| IBIS file stm32g030_031_041_lqfp48.ibs
[IBIS ver] 4.2
[File name] stm32g030_031_041_lqfp48.ibs
[File Rev] rev1.1
[Date]  12-05-2022
[Source] Data Created at STMicroelectronics
[Notes]  File originated from ELDO simulations.
[Disclaimer]  This information is for modeling purpose only and is
   not guaranted. The information is subject to change without
   notice.
[Copyright] Copyright 2022 STMicroelectronics Inc.
|   Component stm32g030_031_041_lqfp48
[Component] stm32g030_031_041_lqfp48
[Manufacturer] STMicroelectronics
[Package]
| variable   typ   min   max
R_pkg   0.0   0.0   0.0
L_pkg   0.0H   0.0H   0.0H
C_pkg   0.0F   0.0F   0.0F
[Pin]   signal_name   model_name  R_pin L_pin C_pin
1 PC13 io8prog2m25m50m120m_sudq_ft 0.053 3.42534E-09 9.041E-14
2 PC14-OSC32_IN io8prog2m25m50m120m_sudq_ft 0.048377332 2.91404E-09 6.443E-14
3 PC15-OSC32_OUT io8prog2m25m50m120m_sudq_ft 0.044678997 2.50442E-09 4.365E-14
4 VBAT POWER 0.041905328 2.19704E-09 2.807E-14
5 VREF+ POWER 0.040056325 1.9919E-09 1.769E-14
6 VDDA POWER 0.03913 1.89021E-09 1.24625E-14
7 VSS GND 0.03913 1.89021E-09 1.24625E-14
8 PF0-OSC_IN io6_ft 0.040057312 1.98992E-09 1.775E-14
9 PF1-OSC_OUT io6_ft 0.041906973 2.19374E-09 2.817E-14
10 PF2-NRST io6reset 0.0446813 2.4998E-09 4.379E-14
11 PA0 io6_ft 0.048380293 2.9081E-09 6.461E-14
12 PA1 io6_ft 0.053 3.42534E-09 9.041E-14
13 PA2 io6_ft 0.053 3.42534E-09 9.041E-14
14 PA3 io6_ft 0.048377332 2.91404E-09 6.443E-14
15 PA4 io6_ft 0.044678997 2.50442E-09 4.365E-14
16 PA5 io6_ft 0.041905328 2.19704E-09 2.807E-14
17 PA6 io6_ft 0.040056325 1.9919E-09 1.769E-14
18 PA7 io6_ft 0.03913 1.89021E-09 1.24625E-14
19 PB0 io6_ft 0.03913 1.89021E-09 1.24625E-14
20 PB1 io6_ft 0.040057312 1.98992E-09 1.775E-14
21 PB2 io6_ft 0.041906973 2.19374E-09 2.817E-14
22 PB10 io6_i2c_ft 0.0446813 2.4998E-09 4.379E-14
23 PB11 io6_i2c_ft 0.048380293 2.9081E-09 6.461E-14
24 PB12 io6_ft 0.053 3.42534E-09 9.041E-14
25 PB13 io6_i2c_ft 0.053 3.42534E-09 9.041E-14
26 PB14 io6_i2c_ft 0.048377332 2.91404E-09 6.443E-14
27 PB15 io6_ft 0.044678997 2.50442E-09 4.365E-14
28 PA8 io6_ft 0.041905328 2.19704E-09 2.807E-14
29 PA9 io6_i2c_ft 0.040056325 1.9919E-09 1.769E-14
30 PC6 io6_ft 0.03913 1.89021E-09 1.24625E-14
31 PC7 io6_ft 0.03913 1.89021E-09 1.24625E-14
32 PA10 io6_i2c_ft 0.040057312 1.98992E-09 1.775E-14
33 PA11 io6_i2c_ft 0.041906973 2.19374E-09 2.817E-14
34 PA12 io6_i2c_ft 0.0446813 2.4998E-09 4.379E-14
35 PA13 io6_ft 0.048380293 2.9081E-09 6.461E-14
36 PA14-BOOT0 io6_ft 0.053 3.42534E-09 9.041E-14
37 PA15 io6_ft 0.053 3.42534E-09 9.041E-14
38 PD0 io6_ft 0.048377332 2.91404E-09 6.443E-14
39 PD1 io6_ft 0.044678997 2.50442E-09 4.365E-14
40 PD2 io6_ft 0.041905328 2.19704E-09 2.807E-14
41 PD3 io6_ft 0.040056325 1.9919E-09 1.769E-14
42 PB3 io6_ft 0.03913 1.89021E-09 1.24625E-14
43 PB4 io6_ft 0.03913 1.89021E-09 1.24625E-14
44 PB5 io6_ft 0.040057312 1.98992E-09 1.775E-14
45 PB6 io6_i2c_ft 0.041906973 2.19374E-09 2.817E-14
46 PB7 io6_i2c_ft 0.0446813 2.4998E-09 4.379E-14
47 PB8 io6_i2c_ft 0.048380293 2.9081E-09 6.461E-14
48 PB9 io6_i2c_ft 0.053 3.42534E-09 9.041E-14
[Model Selector] io8prog2m25m50m120m_sudq_ft
iols8p_sudq_ft_pd_lv  "IO low speed, PD=40kOhm - 1P8V"
iols8p_sudq_ft_pu_lv  "IO low speed, PU=40kOhm - 1P8V"
iols8p_sudq_ft_lv  "IO low speed - 1P8V"
iols8p_sudq_ft_pd  "IO low speed, PD=40kOhm - 3P3V"
iols8p_sudq_ft_pu  "IO low speed, PU=40kOhm - 3P3V"
iols8p_sudq_ft  "IO low speed - 3P3V"
iofs8p_sudq_ft_pd_lv  "IO full speed, PD=40kOhm - 1P8V"
iofs8p_sudq_ft_pu_lv  "IO full speed, PU=40kOhm - 1P8V"
iofs8p_sudq_ft_lv  "IO full speed - 1P8V"
iofs8p_sudq_ft_pd  "IO full speed, PD=40kOhm - 3P3V"
iofs8p_sudq_ft_pu  "IO full speed, PU=40kOhm - 3P3V"
iofs8p_sudq_ft  "IO full speed - 3P3V"
ioms8p_sudq_ft_pd_lv  "IO medium speed, PD=40kOhm - 1P8V"
ioms8p_sudq_ft_pu_lv  "IO medium speed, PU=40kOhm - 1P8V"
ioms8p_sudq_ft_lv  "IO medium speed - 1P8V"
ioms8p_sudq_ft_pd  "IO medium speed, PD=40kOhm - 3P3V"
ioms8p_sudq_ft_pu  "IO medium speed, PU=40kOhm - 3P3V"
ioms8p_sudq_ft  "IO medium speed - 3P3V"
iohs8p_sudq_ft_pd_lv  "IO high speed, PD=40kOhm - 1P8V"
iohs8p_sudq_ft_pu_lv  "IO high speed, PU=40kOhm - 1P8V"
iohs8p_sudq_ft_lv  "IO high speed - 1P8V"
iohs8p_sudq_ft_pd  "IO high speed, PD=40kOhm - 3P3V"
iohs8p_sudq_ft_pu  "IO high speed, PU=40kOhm - 3P3V"
iohs8p_sudq_ft  "IO high speed - 3P3V"
[Model Selector] io6_ft
io6_ft_1v8_highspeed_pd  "GPIO-1.8V range - high speed - pull down"
io6_ft_1v8_fastspeed_pd  "GPIO-1.8V range - fast speed - pull down"
io6_ft_1v8_mediumspeed_pd  "GPIO-1.8V range - medium speed - pull down"
io6_ft_1v8_lowspeed_pd  "GPIO-1.8V range - low speed - pull down"
io6_ft_1v8_highspeed_pu  "GPIO-1.8V range - high speed - pull up"
io6_ft_1v8_fastspeed_pu  "GPIO-1.8V range - fast speed - pull up"
io6_ft_1v8_mediumspeed_pu  "GPIO-1.8V range - medium speed - pull up"
io6_ft_1v8_lowspeed_pu  "GPIO-1.8V range - low speed - pull up"
io6_ft_1v8_highspeed  "GPIO-1.8V range - high speed"
io6_ft_1v8_fastspeed  "GPIO-1.8V range - fast speed"
io6_ft_1v8_mediumspeed  "GPIO-1.8V range - medium speed"
io6_ft_1v8_lowspeed  "GPIO-1.8V range - low speed"
io6_ft_3v3_highspeed_pd  "GPIO-3.3V range - high speed - pull down"
io6_ft_3v3_fastspeed_pd  "GPIO-3.3V range - fast speed - pull down"
io6_ft_3v3_mediumspeed_pd  "GPIO-3.3V range - medium speed - pull down"
io6_ft_3v3_lowspeed_pd  "GPIO-3.3V range - low speed - pull down"
io6_ft_3v3_highspeed_pu  "GPIO-3.3V range - high speed - pull up"
io6_ft_3v3_fastspeed_pu  "GPIO-3.3V range - fast speed - pull up"
io6_ft_3v3_mediumspeed_pu  "GPIO-3.3V range - medium speed - pull up"
io6_ft_3v3_lowspeed_pu  "GPIO-3.3V range - low speed - pull up"
io6_ft_3v3_highspeed  "GPIO-3.3V range - high speed"
io6_ft_3v3_fastspeed  "GPIO-3.3V range - fast speed"
io6_ft_3v3_mediumspeed  "GPIO-3.3V range - medium speed"
io6_ft_3v3_lowspeed  "GPIO-3.3V range - low speed"
[Model Selector] io6_i2c_ft
io6_ft_1v8_highspeed_pd  "GPIO-1.8V range - high speed - pull down"
io6_ft_1v8_fastspeed_pd  "GPIO-1.8V range - fast speed - pull down"
io6_ft_1v8_mediumspeed_pd  "GPIO-1.8V range - medium speed - pull down"
io6_ft_1v8_lowspeed_pd  "GPIO-1.8V range - low speed - pull down"
io6_ft_1v8_highspeed_pu  "GPIO-1.8V range - high speed - pull up"
io6_ft_1v8_fastspeed_pu  "GPIO-1.8V range - fast speed - pull up"
io6_ft_1v8_mediumspeed_pu  "GPIO-1.8V range - medium speed - pull up"
io6_ft_1v8_lowspeed_pu  "GPIO-1.8V range - low speed - pull up"
io6_ft_1v8_highspeed  "GPIO-1.8V range - high speed"
io6_ft_1v8_fastspeed  "GPIO-1.8V range - fast speed"
io6_ft_1v8_mediumspeed  "GPIO-1.8V range - medium speed"
io6_ft_1v8_lowspeed  "GPIO-1.8V range - low speed"
io6_ft_3v3_highspeed_pd  "GPIO-3.3V range - high speed - pull down"
io6_ft_3v3_fastspeed_pd  "GPIO-3.3V range - fast speed - pull down"
io6_ft_3v3_mediumspeed_pd  "GPIO-3.3V range - medium speed - pull down"
io6_ft_3v3_lowspeed_pd  "GPIO-3.3V range - low speed - pull down"
io6_ft_3v3_highspeed_pu  "GPIO-3.3V range - high speed - pull up"
io6_ft_3v3_fastspeed_pu  "GPIO-3.3V range - fast speed - pull up"
io6_ft_3v3_mediumspeed_pu  "GPIO-3.3V range - medium speed - pull up"
io6_ft_3v3_lowspeed_pu  "GPIO-3.3V range - low speed - pull up"
io6_ft_3v3_highspeed  "GPIO-3.3V range - high speed"
io6_ft_3v3_fastspeed  "GPIO-3.3V range - fast speed"
io6_ft_3v3_mediumspeed  "GPIO-3.3V range - medium speed"
io6_ft_3v3_lowspeed  "GPIO-3.3V range - low speed"
io6_ft_1v8_highi2c_pd   "GPIO-1.8V range - high   speed i2c mode - pd"
io6_ft_1v8_fasti2c_pd   "GPIO-1.8V range - fast   speed i2c mode - pd"
io6_ft_1v8_mediumi2c_pd  "GPIO-1.8V range - medium speed i2c mode - pd"
io6_ft_1v8_lowi2c_pd   "GPIO-1.8V range - low   speed i2c mode - pd"
io6_ft_1v8_highi2c_pu   "GPIO-1.8V range - high   speed i2c mode - pu"
io6_ft_1v8_fasti2c_pu   "GPIO-1.8V range - fast   speed i2c mode - pu"
io6_ft_1v8_mediumi2c_pu  "GPIO-1.8V range - medium speed i2c mode - pu"
io6_ft_1v8_lowi2c_pu   "GPIO-1.8V range - low   speed i2c mode - pu"
io6_ft_1v8_highi2c   "GPIO-1.8V range - high   speed i2c mode"
io6_ft_1v8_fasti2c   "GPIO-1.8V range - fast   speed i2c mode"
io6_ft_1v8_mediumi2c   "GPIO-1.8V range - medium speed i2c mode"
io6_ft_1v8_lowi2c   "GPIO-1.8V range - low   speed i2c mode"
io6_ft_3v3_highi2c_pd   "GPIO-3.3V range - high   speed i2c mode - pd"
io6_ft_3v3_fasti2c_pd   "GPIO-3.3V range - fast   speed i2c mode - pd"
io6_ft_3v3_mediumi2c_pd  "GPIO-3.3V range - medium speed i2c mode - pd"
io6_ft_3v3_lowi2c_pd   "GPIO-3.3V range - low   speed i2c mode - pd"
io6_ft_3v3_highi2c_pu   "GPIO-3.3V range - high   speed i2c mode - pu"
io6_ft_3v3_fasti2c_pu   "GPIO-3.3V range - fast   speed i2c mode - pu"
io6_ft_3v3_mediumi2c_pu  "GPIO-3.3V range - medium speed i2c mode - pu"
io6_ft_3v3_lowi2c_pu   "GPIO-3.3V range - low   speed i2c mode - pu"
io6_ft_3v3_highi2c   "GPIO-3.3V range - high   speed i2c mode"
io6_ft_3v3_fasti2c   "GPIO-3.3V range - fast   speed i2c mode"
io6_ft_3v3_mediumi2c   "GPIO-3.3V range - medium speed i2c mode"
io6_ft_3v3_lowi2c   "GPIO-3.3V range - low   speed i2c mode"
io6_i2c_ft_1v8_pd  "GPIO-1.8V I2C fm+ - pd"
io6_i2c_ft_3v3_pd  "GPIO-3.3V I2C fm+ - pd"
io6_i2c_ft_1v8_pu  "GPIO-1.8V I2C fm+ - pu"
io6_i2c_ft_3v3_pu  "GPIO-3.3V I2C fm+ - pu"
io6_i2c_ft_1v8   "GPIO-1.8V I2C fm+"
io6_i2c_ft_3v3   "GPIO-3.3V I2C fm+"
[Model Selector] io6reset
io6_ft_1v8_highspeed_pd  "GPIO-1.8V range - high speed - pull down"
io6_ft_1v8_fastspeed_pd  "GPIO-1.8V range - fast speed - pull down"
io6_ft_1v8_mediumspeed_pd  "GPIO-1.8V range - medium speed - pull down"
io6_ft_1v8_lowspeed_pd  "GPIO-1.8V range - low speed - pull down"
io6_ft_1v8_highspeed_pu  "GPIO-1.8V range - high speed - pull up"
io6_ft_1v8_fastspeed_pu  "GPIO-1.8V range - fast speed - pull up"
io6_ft_1v8_mediumspeed_pu  "GPIO-1.8V range - medium speed - pull up"
io6_ft_1v8_lowspeed_pu  "GPIO-1.8V range - low speed - pull up"
io6_ft_1v8_highspeed  "GPIO-1.8V range - high speed"
io6_ft_1v8_fastspeed  "GPIO-1.8V range - fast speed"
io6_ft_1v8_mediumspeed  "GPIO-1.8V range - medium speed"
io6_ft_1v8_lowspeed  "GPIO-1.8V range - low speed"
io6_ft_3v3_highspeed_pd  "GPIO-3.3V range - high speed - pull down"
io6_ft_3v3_fastspeed_pd  "GPIO-3.3V range - fast speed - pull down"
io6_ft_3v3_mediumspeed_pd  "GPIO-3.3V range - medium speed - pull down"
io6_ft_3v3_lowspeed_pd  "GPIO-3.3V range - low speed - pull down"
io6_ft_3v3_highspeed_pu  "GPIO-3.3V range - high speed - pull up"
io6_ft_3v3_fastspeed_pu  "GPIO-3.3V range - fast speed - pull up"
io6_ft_3v3_mediumspeed_pu  "GPIO-3.3V range - medium speed - pull up"
io6_ft_3v3_lowspeed_pu  "GPIO-3.3V range - low speed - pull up"
io6_ft_3v3_highspeed  "GPIO-3.3V range - high speed"
io6_ft_3v3_fastspeed  "GPIO-3.3V range - fast speed"
io6_ft_3v3_mediumspeed  "GPIO-3.3V range - medium speed"
io6_ft_3v3_lowspeed  "GPIO-3.3V range - low speed"
ioreset_1v2_pu  "RESET 1.2V range with PU"
ioreset_1v2  "RESET 1.2V range"
ioreset_1v8_pu  "RESET 1.8V range with PU"
ioreset_1v8  "RESET 1.8V range"
ioreset_3v3_pu  "RESET 3.3V range with PU"
ioreset_3v3  "RESET 3.3V range"
| Models and submodels in the file (84): iols8p_sudq_ft_pd_lv (I/O), iols8p_sudq_ft_pu_lv (I/O), iols8p_sudq_ft_lv (I/O), iols8p_sudq_ft_pd (I/O), iols8p_sudq_ft_pu (I/O), iols8p_sudq_ft (I/O), iofs8p_sudq_ft_pd_lv (I/O), iofs8p_sudq_ft_pu_lv (I/O), iofs8p_sudq_ft_lv (I/O), iofs8p_sudq_ft_pd (I/O), iofs8p_sudq_ft_pu (I/O), iofs8p_sudq_ft (I/O), ioms8p_sudq_ft_pd_lv (I/O), ioms8p_sudq_ft_pu_lv (I/O), ioms8p_sudq_ft_lv (I/O), ioms8p_sudq_ft_pd (I/O), ioms8p_sudq_ft_pu (I/O), ioms8p_sudq_ft (I/O), iohs8p_sudq_ft_pd_lv (I/O), iohs8p_sudq_ft_pu_lv (I/O), iohs8p_sudq_ft_lv (I/O), iohs8p_sudq_ft_pd (I/O), iohs8p_sudq_ft_pu (I/O), iohs8p_sudq_ft (I/O), io6_ft_1v8_highspeed_pd (I/O), io6_ft_1v8_fastspeed_pd (I/O), io6_ft_1v8_mediumspeed_pd (I/O), io6_ft_1v8_lowspeed_pd (I/O), io6_ft_1v8_highspeed_pu (I/O), io6_ft_1v8_fastspeed_pu (I/O), io6_ft_1v8_mediumspeed_pu (I/O), io6_ft_1v8_lowspeed_pu (I/O), io6_ft_1v8_highspeed (I/O), io6_ft_1v8_fastspeed (I/O), io6_ft_1v8_mediumspeed (I/O), io6_ft_1v8_lowspeed (I/O), io6_ft_3v3_highspeed_pd (I/O), io6_ft_3v3_fastspeed_pd (I/O), io6_ft_3v3_mediumspeed_pd (I/O), io6_ft_3v3_lowspeed_pd (I/O), io6_ft_3v3_highspeed_pu (I/O), io6_ft_3v3_fastspeed_pu (I/O), io6_ft_3v3_mediumspeed_pu (I/O), io6_ft_3v3_lowspeed_pu (I/O), io6_ft_3v3_highspeed (I/O), io6_ft_3v3_fastspeed (I/O), io6_ft_3v3_mediumspeed (I/O), io6_ft_3v3_lowspeed (I/O), io6_i2c_ft_1v8_pd (I/O_open_drain), io6_i2c_ft_3v3_pd (I/O_open_drain), io6_i2c_ft_1v8_pu (I/O_open_drain), io6_i2c_ft_3v3_pu (I/O_open_drain), io6_i2c_ft_1v8 (I/O_open_drain), io6_i2c_ft_3v3 (I/O_open_drain), io6_ft_1v8_highi2c_pd (I/O_open_drain), io6_ft_1v8_fasti2c_pd (I/O_open_drain), io6_ft_1v8_mediumi2c_pd (I/O_open_drain), io6_ft_1v8_lowi2c_pd (I/O_open_drain), io6_ft_1v8_highi2c_pu (I/O_open_drain), io6_ft_1v8_fasti2c_pu (I/O_open_drain), io6_ft_1v8_mediumi2c_pu (I/O_open_drain), io6_ft_1v8_lowi2c_pu (I/O_open_drain), io6_ft_1v8_highi2c (I/O_open_drain), io6_ft_1v8_fasti2c (I/O_open_drain), io6_ft_1v8_mediumi2c (I/O_open_drain), io6_ft_1v8_lowi2c (I/O_open_drain), io6_ft_3v3_highi2c_pd (I/O_open_drain), io6_ft_3v3_fasti2c_pd (I/O_open_drain), io6_ft_3v3_mediumi2c_pd (I/O_open_drain), io6_ft_3v3_lowi2c_pd (I/O_open_drain), io6_ft_3v3_highi2c_pu (I/O_open_drain), io6_ft_3v3_fasti2c_pu (I/O_open_drain), io6_ft_3v3_mediumi2c_pu (I/O_open_drain), io6_ft_3v3_lowi2c_pu (I/O_open_drain), io6_ft_3v3_highi2c (I/O_open_drain), io6_ft_3v3_fasti2c (I/O_open_drain), io6_ft_3v3_mediumi2c (I/O_open_drain), io6_ft_3v3_lowi2c (I/O_open_drain), ioreset_1v2_pu (I/O_open_drain), ioreset_1v2 (I/O_open_drain)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
